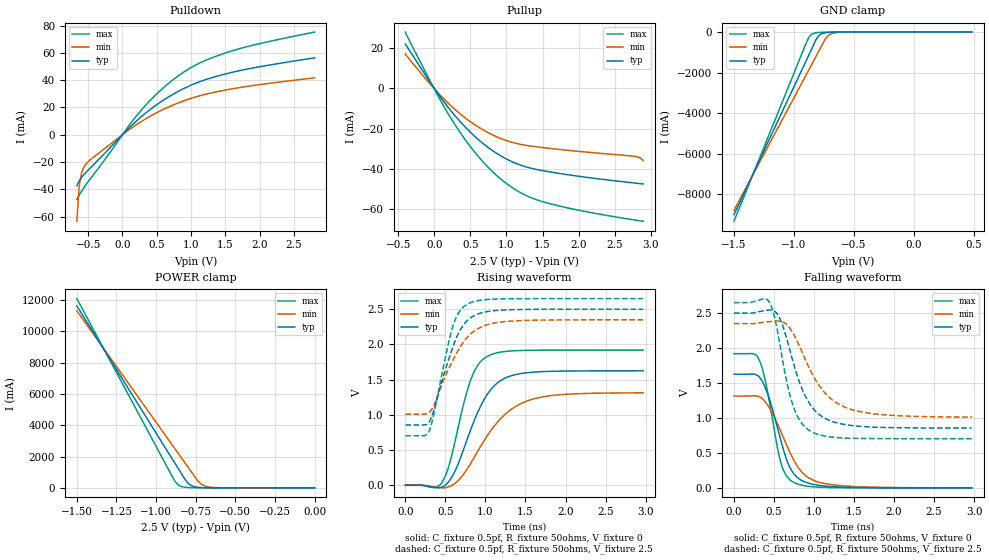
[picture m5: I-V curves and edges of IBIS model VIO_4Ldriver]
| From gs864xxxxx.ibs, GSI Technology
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|  signals   DQA1-DQA9, DQB1-DQB9, DQC1-DQC9, DQD1-DQD9
[Model]   VIO_4Ldriver
Model_type   I/O
Polarity   Non-Inverting
Vinl  =   0.75v
Vinh  =   1.75v
Vmeas =   1.25v
Cref  =   0pF
Rref  =   50
Vref  =   1.25v
|  variable   typ   min   max
C_comp   3.0pF   2.5pF   3.5pF
|  variable   typ   min   max
[Temperature Range]   50   0   100
|  variable   typ   min   max
[Voltage Range]   2.5   2.35   2.65
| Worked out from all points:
|   slope of the pulldown table from 0 to 0.375 V, typ, clamps not added: 21.6 ohm
|   slope of the pullup table from 0 to 0.375 V, typ, clamps not added: 21.9 ohm
|   GND clamp passes 1 mA (typ) near -0.58 V on its own axis
|   POWER clamp passes 1 mA (typ) near -0.61 V on its own axis
|   rising waveform, C_fixture 0.5pf, R_fixture 50ohms, V_fixture 0: 20-80 % time 362ps typ, 501ps min, 259ps max; typ from 0 V to 1.62 V
|   rising waveform, C_fixture 0.5pf, R_fixture 50ohms, V_fixture 2.5: 20-80 % time 284ps typ, 353ps min, 224ps max; typ from 0.855 V to 2.5 V
|   falling waveform, C_fixture 0.5pf, R_fixture 50ohms, V_fixture 0: 20-80 % time 252ps typ, 334ps min, 189ps max; typ from 1.62 V to 0 V
|   falling waveform, C_fixture 0.5pf, R_fixture 50ohms, V_fixture 2.5: 20-80 % time 307ps typ, 410ps min, 225ps max; typ from 2.5 V to 0.856 V
[Pulldown]
| voltage   typ   min   max
-665mV    -37.48mA   -63.5mA    -47.42mA
-630mV    -33.87mA   -37.7mA    -44.28mA
-595mV    -31.34mA   -27.86mA   -41.36mA
-560mV    -29.22mA   -23.52mA   -38.66mA
-385mV    -20.1mA    -15.04mA   -26.82mA
105mV     5.397mA    3.94mA     7.392mA
315mV     14.92mA    10.93mA    20.35mA
525mV     22.94mA    16.83mA    31.19mA
770mV     30.61mA    22.48mA    41.55mA
1.19V     40.05mA    29.41mA    54.09mA
1.785V    47.84mA    35.21mA    64.23mA
2.8V      56.39mA    41.84mA    75.34mA
[Pullup]
| voltage (VDDQ-Vout) typ   min   max
-400mV    21.9mA     17.14mA    27.88mA
25mV      -1.299mA   -1.191mA   -2.024mA
305mV     -14.32mA   -11.03mA   -19.02mA
480mV     -21.05mA   -16.03mA   -27.95mA
655mV     -26.75mA   -20.17mA   -35.62mA
970mV     -34.47mA   -25.52mA   -46.36mA
1.25V     -38.71mA   -28.14mA   -52.74mA
1.53V     -40.98mA   -29.49mA   -56.47mA
2.02V     -43.68mA   -31.32mA   -60.56mA
2.755V    -46.86mA   -33.62mA   -65.13mA
2.825V    -47.14mA   -34.08mA   -65.52mA
2.895V    -47.42mA   -35.78mA   -65.9mA
[GND Clamp]
| voltage   typ   min   max
-1.5V     -9.007A    -8.796A    -9.334A
-900mV    -1.426A    -2.122A    -562.9mA
-880mV    -1.174A    -1.9A      -292.9mA
-860mV    -921.1mA   -1.678A    -142.5mA
-820mV    -416.2mA   -1.233A    -38.58mA
-800mV    -222mA     -1.011A    -23.51mA
-780mV    -116.3mA   -788.8mA   -16.2mA
-740mV    -33.04mA   -348.7mA   -9.876mA
-720mV    -18.57mA   -198.2mA   -8.142mA
-700mV    -10.99mA   -111mA     -6.744mA
-660mV    -4.5mA     -34.67mA   -4.472mA
480mV     -174.2pA   381.8pA    -282pA
[POWER Clamp]
| voltage (VDDQ-Vout) typ   min   max
-1.5V     11.62A     11.31A     12.09A
-900mV    1.877A     2.768A     763.5mA
-880mV    1.553A     2.483A     398.4mA
-860mV    1.228A     2.198A     183.4mA
-840mV    903.6mA    1.913A     83.63mA
-800mV    304.2mA    1.344A     19.44mA
-780mV    154.7mA    1.059A     10.68mA
-740mV    39.51mA    489.9mA    4.639mA
-720mV    20.32mA    274.5mA    3.532mA
-680mV    5.894mA    82.85mA    2.298mA
-580mV    568.7uA    4.201mA    684.1uA
0V        773.3pA    2.256nA    488.4pA
[Ramp]
| voltage   typ   min   max
dV/dt_r   1.53/137p   1.35/170p   1.77/112p
dV/dt_f   1.51/136p   1.31/167p   1.77/112p
R_load  =   50ohms
[Rising Waveform]
C_fixture =   0.5pf
R_fixture =   50ohms
V_fixture =   0
| Time   V(typ)   V(min)   V(max)
0s        7.126nV    16.14nV    4.94nV
450ps     -30.66mV   -35.47mV   25.66mV
510ps     12.66mV    -32.07mV   160.6mV
600ps     156.9mV    10.68mV    522.6mV
810ps     774.5mV    302mV      1.48V
930ps     1.1V       534.8mV    1.744V
1.02ns    1.288V     699.5mV    1.828V
1.26ns    1.529V     1.022V     1.901V
1.62ns    1.608V     1.232V     1.917V
2.97ns    1.625V     1.312V     1.919V
[Rising Waveform]
C_fixture =   0.5pf
R_fixture =   50ohms
V_fixture =   2.5
V_fixture_min =   2.35
V_fixture_max =   2.65
| Time   V(typ)   V(min)   V(max)
0s        855.1mV    1.009V     703mV
240ps     854.5mV    1.008V     703.2mV
300ps     902mV      1.035V     774.3mV
540ps     1.786V     1.655V     2.029V
600ps     1.987V     1.79V      2.286V
690ps     2.217V     1.974V     2.489V
780ps     2.346V     2.109V     2.576V
960ps     2.451V     2.253V     2.631V
1.23ns    2.488V     2.322V     2.647V
2.97ns    2.5V       2.35V      2.65V
[Falling Waveform]
C_fixture =   0.5pf
R_fixture =   50ohms
V_fixture =   0
| Time   V(typ)   V(min)   V(max)
0s        1.625V     1.313V     1.919V
240ps     1.628V     1.317V     1.919V
330ps     1.567V     1.296V     1.791V
390ps     1.433V     1.232V     1.54V
570ps     744.1mV    845mV      426.5mV
630ps     498.3mV    684.6mV    220mV
720ps     247.5mV    455.1mV    95.37mV
900ps     78.1mV     168.9mV    26.32mV
1.14ns    25.11mV    60.34mV    5.392mV
2.97ns    11.45uV    292.8uV    -191.8nV
[Falling Waveform]
C_fixture =   0.5pf
R_fixture =   50ohms
V_fixture =   2.5
V_fixture_min =   2.35
V_fixture_max =   2.65
| Time   V(typ)   V(min)   V(max)
0s        2.5V       2.35V      2.65V
450ps     2.546V     2.378V     2.639V
510ps     2.524V     2.385V     2.433V
570ps     2.43V      2.384V     2.07V
720ps     1.875V     2.246V     1.239V
840ps     1.444V     1.969V     931.6mV
960ps     1.177V     1.667V     808.6mV
1.2ns     960.8mV    1.284V     728.9mV
1.5ns     887.7mV    1.11V      708mV
2.97ns    855.5mV    1.012V     703.1mV
